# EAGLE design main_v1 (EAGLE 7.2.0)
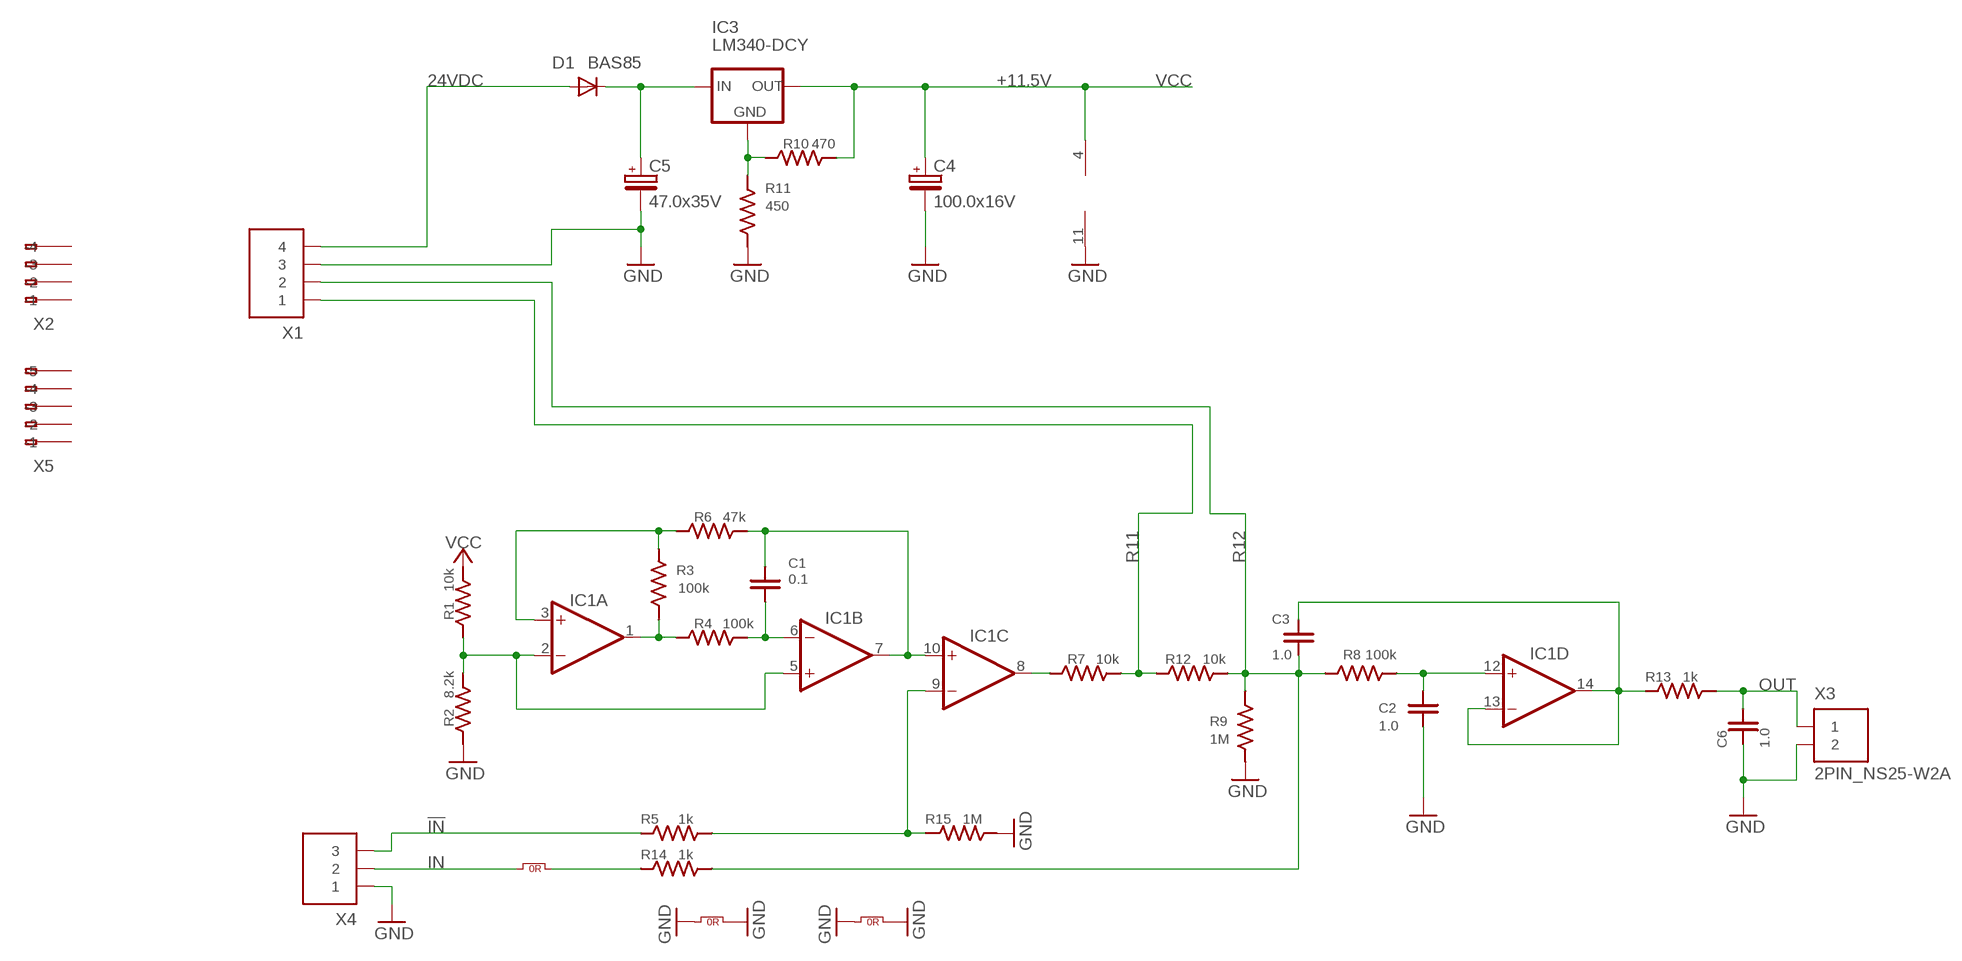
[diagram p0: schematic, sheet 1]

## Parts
C1  0.1  C/0805  [C0805]
C2  1.0  C/0805  [C0805]
C3  1.0  C/0805  [C0805]
C4  100.0x16V  CPOL-EUSANYO_SMD_C6  [SANYO-OSCON_SMD_C6]
C5  47.0x35V  CPOL-EUSANYO_SMD_C6  [SANYO-OSCON_SMD_C6]
C6  1.0  C/0805  [C0805]
D1  BAS85  DIODE-MINIMELF  [MINIMELF]
IC1  LM2902D  [SO14]
IC3  LM340-DCY  LM340MP-5V-DCY  [SOT223]
J1  0R  JUMPER  [R0805]
J2  0R  JUMPER  [R0805]
J3  0R  JUMPER  [R0805]
R1  10k  R/0805  [R0805]
R2  8.2k  R/0805  [R0805]
R3  100k  R/0805  [R0805]
R4  100k  R/0805  [R0805]
R5  1k  R/0805  [R0805]
R6  47k  R/0805  [R0805]
R7  10k  R/0805  [R0805]
R8  100k  R/0805  [R0805]
R9  1M  R/0805  [R0805]
R10  470  R/0805  [R0805]
R11  450  R/0805  [R0805]
R12  10k  R/0805  [R0805]
R13  1k  R/0805  [R0805]
R14  1k  R/0805  [R0805]
R15  1M  R/0805  [R0805]
X1  4PIN_NS25-W4A  [7395-04]
X2  233-104  [233-104]
X3  2PIN_NS25-W2A  [7395-02]
X4  3PIN_NS25-W3A  [7395-03]
X5  233-105  [233-105]

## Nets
24VDC [power]: D1.A X1.4
!IN!: R5.1 X4.3
GND: C2.1 C4.- C5.- C6.1 IC1.11(P:V-) J2.1 J2.2 J3.1 J3.2 R2.1 R9.1 R11.1 R15.1 X1.3 X3.2 X4.1
IN: J1.1 X4.2
N$1: IC1.2(A:-IN) IC1.5(B:+IN) R1.1 R2.2
N$2: IC1.3(A:+IN) R3.1 R6.1
N$3: IC1.8(C:OUT) R7.1
N$4: C1.1 IC1.6(B:-IN) R4.2
N$5: IC1.1(A:OUT) R3.2 R4.1
N$6: J1.2 R14.1
N$7: C1.2 IC1.7(B:OUT) IC1.10(C:+IN) R6.2
N$8: IC1.9(C:-IN) R5.2 R15.2
N$9: C2.2 IC1.12(D:+IN) R8.2
N$10: C3.2 IC1.13(D:-IN) IC1.14(D:OUT) R13.1
N$11: IC3.2(GND) IC3.4(GND) R10.1 R11.2
N$13 [power]: C5.+ D1.C IC3.1(IN)
OUT: C6.2 R13.2 X3.1
R11: R7.2 R12.1 X1.1
R12: C3.1 R8.1 R9.2 R12.2 R14.2 X1.2
VCC [power]: C4.+ IC1.4(P:V+) IC3.3(OUT) R1.2 R10.2
Unconnected: X2.A1(-1) X2.A2(-2) X2.A3(-3) X2.A4(-4) X2.B1(B-1) X2.B2(B-2) X2.B3(B-3) X2.B4(B-4) X5.A1(-1) X5.A2(-2) X5.A3(-3) X5.A4(-4) X5.A5(-5) X5.B1(B-1) X5.B2(B-2) X5.B3(B-3) X5.B4(B-4) X5.B5(B-5)

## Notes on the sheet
- +11.5V

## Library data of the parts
C1-C3 C6 = descreet:C
C4 C5 = rcl:CPOL-EU: POLARIZED CAPACITOR, European symbol
D1 = diode:DIODE-: DIODE
IC1 = linear:LM2902: COMPARATOR
IC3 = touch:LM340*
J1-J3 = smd-special:JUMPER
R1-R15 = descreet:R
X1 = connectors:4PIN_
X2 = con-wago:233-104: WAGO Cage Clamp
X3 = connectors:2PIN_
X4 = connectors:3PIN_
X5 = con-wago:233-105: WAGO Cage Clamp

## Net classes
0 default: clearance 0.205 mm
1 power: clearance 0.3 mm

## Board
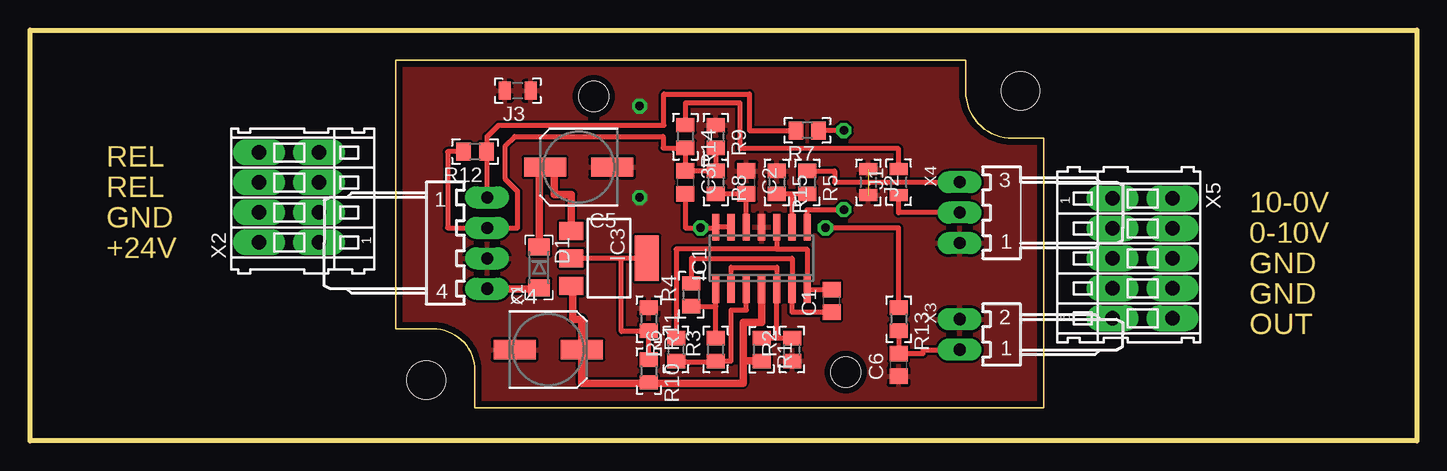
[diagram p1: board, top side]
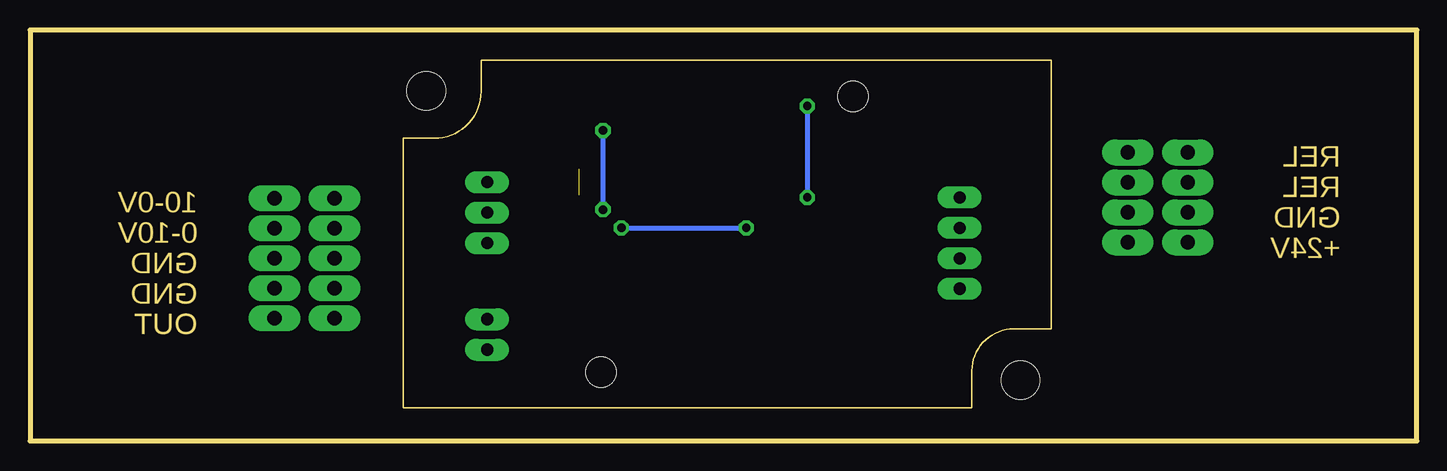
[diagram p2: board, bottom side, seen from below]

Size 115.57 x 34.29 mm. Coordinates in mm from the lower left corner, seen from the top.
Outline: 0,34.29 115.57,34.29 115.57,0 0,0 0,34.29
Copper layers (1*16): Top 0.035mm / dielectric 1.5mm / Bottom 0.035mm
Design rules "default *": minimum track width 10mil, minimum drill 24mil, track to track 8mil, track to pad 8mil, pad to pad 8mil, via to via 8mil, smd to smd 8mil, copper to edge 20mil, drill to drill 8mil, minimum pad ring 10mil, minimum via ring 8mil, stop-mask expansion 4mil, vias tented up to drill 0mil, thermal gap 10mil
Holes 3.2 mm at 33.02,5.08 82.55,29.21

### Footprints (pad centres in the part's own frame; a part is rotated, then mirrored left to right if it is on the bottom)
C0805 = smd 1.3 x 1.5: 1 -0.95,0; 2 0.95,0
SANYO-OSCON_SMD_C6 = smd 3.5 x 1.6: + 2.8,0; - -2.8,0
MINIMELF = smd 1.4 x 1.8: A 1.7,0; C -1.7,0
SO14 = smd 0.6 x 2.2: 1 -3.81,-2.6; 2 -2.54,-2.6; 3 -1.27,-2.6; 4 0,-2.6; 5 1.27,-2.6; 6 2.54,-2.6; 7 3.81,-2.6; 8 3.81,2.6; 9 2.54,2.6; 10 1.27,2.6; 11 0,2.6; 12 -1.27,2.6; 13 -2.54,2.6; 14 -3.81,2.6
SOT223 = smd 1.5 x 2: 1 -2.3,-3.15; 2 0,-3.15; 3 2.3,-3.15 | smd 3.8 x 2: 4 0,3.15
R0805 = smd 1 x 1.5: 1 -1.077,0; 2 1.077,0
R0805' = smd 1.2 x 1.5: 1 -0.95,0; 2 0.95,0
1551H = hole 2.5: 16.5,-3; 37.5,-26
7395-04 = drill 1.016 long: 1 -3.81,0; 2 -1.27,0; 3 1.27,0; 4 3.81,0
233-104 = drill 1.2 long: A1 -3.75,2.5; A2 -1.25,2.5; A3 1.25,2.5; A4 3.75,2.5; B1 -3.75,-2.5; B2 -1.25,-2.5; B3 1.25,-2.5; B4 3.75,-2.5
7395-02 = drill 1.016 long: 1 -1.27,0; 2 1.27,0
7395-03 = drill 1.016 long: 1 -2.54,0; 2 0,0; 3 2.54,0
233-105 = drill 1.2 long: A1 -5,2.5; A2 -2.5,2.5; A3 0,2.5; A4 2.5,2.5; A5 5,2.5; B1 -5,-2.5; B2 -2.5,-2.5; B3 0,-2.5; B4 2.5,-2.5; B5 5,-2.5

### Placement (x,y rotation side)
C1  66.8,11.68 90 top
C2  59.69,21.59 270 top
C3  54.61,21.59 270 top
C4  43.18,7.62 0 top
C5  45.72,22.86 180 top
C6  72.39,6.35 90 top
D1  42.42,14.48 270 top
IC1  60.96,15.24 0 top
IC3  48.26,15.24 270 top
J1  72.39,21.59 90 top
J2  69.85,21.59 270 top
J3  40.64,29.21 180 top
R1  10k  [R0805']  60.96,7.62 270 top
R2  8.2k  [R0805']  63.5,7.62 90 top
R3  100k  [R0805']  57.15,7.62 90 top
R4  100k  [R0805']  55.12,12.19 90 top
R5  1k  [R0805']  64.77,21.59 270 top
R6  47k  [R0805']  53.85,7.62 90 top
R7  10k  [R0805']  64.77,25.91 180 top
R8  100k  [R0805']  57.15,21.59 270 top
R9  1M  [R0805']  57.15,25.4 270 top
R10  470  [R0805']  51.56,5.84 270 top
R11  450  [R0805']  51.56,10.16 270 top
R12  10k  [R0805']  37.08,24.13 180 top
R13  1k  [R0805']  72.39,10.16 270 top
R14  1k  [R0805']  54.61,25.4 270 top
R15  1M  [R0805']  62.23,21.59 270 top
U$1  [1551H]  30.48,31.75 0 top
X1  38.1,16.51 270 top
X2  21.59,20.32 90 top
X3  77.47,8.89 90 top
X4  77.47,19.05 90 top
X5  92.71,15.24 270 top

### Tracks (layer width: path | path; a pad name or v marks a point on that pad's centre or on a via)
24VDC
  Top 0.406: 42.42,12.7 D1.A
  Top 0.61: X1.4 42.42,12.7
!IN!
  Top 0.406: X4.3 67.06,21.59 67.06,22.54 R5.1
GND  (via drill 0.7)  (1 unrouted)
  Bottom 0.406: v50.8,27.94 v50.8,20.32
  pour Top: 30.48,31.75 84.33,31.75 84.33,2.79 30.48,2.79
IN
  Top 0.406: X4.2 72.39,19.05 J1.1
N$1
  Top 0.406: R2.2 62.23,8.57 | IC1.2 58.42,14.48 62.23,14.48 IC1.5 62.23,8.57 | 62.23,8.57 R1.1
N$2
  Top 0.406: IC1.3 59.69,10.92 58.42,10.92 58.42,6.67 R3.1 57.15,6.6 54.61,6.6 R6.1
N$3  (via drill 0.7)
  Top 0.406: IC1.8 64.77,19.3 v67.82,19.3 | v67.82,25.91 R7.1
  Bottom 0.406: v67.82,19.3 v67.82,25.91
N$4
  Top 0.406: C1.1 63.5,10.73 IC1.6 63.5,15.24 55.12,15.24 R4.2
N$5
  Top 0.406: R3.2 57.15,11.24 | 57.15,11.24 IC1.1 | R4.1 57.15,11.24
N$6
  Top 0.406: J1.2 72.39,24.38 59.18,24.38 59.18,28.19 54.61,28.19 R14.1
N$7
  Top 0.406: IC1.10 62.23,16 | 62.23,16 64.77,16 IC1.7 C1.2 | 62.23,16 53.85,16 R6.2
N$8
  Top 0.406: R15.2 63.5,20.64 | 63.5,20.64 R5.2 | IC1.9 63.5,20.64
N$9
  Top 0.406: IC1.12 C2.2 R8.2
N$10  (via drill 0.7)
  Top 0.406: IC1.13 IC1.14 57.15,17.78 v55.88,17.78 54.61,17.78 C3.2 | R13.1 72.39,17.78 v66.29,17.78
  Bottom 0.406: v66.29,17.78 v55.88,17.78
N$11
  Top 0.406: IC3.4 49.28,15.24 | 49.28,15.24 IC3.2 | R10.1 R11.2 51.56,9.14 49.28,9.14 49.28,15.24
N$13
  Top 0.406: C5.+ 43.18,22.86 | 45.11,17.53 IC3.1
  Top 0.61: D1.C 42.42,22.36 C5.+ 43.69,22.86 43.69,20.57 45.11,20.57 IC3.1
OUT
  Top 0.406: R13.2 C6.2 74.42,7.3 74.42,7.62 X3.1
R11
  Top 0.406: X1.1 38.1,24.13 | 38.1,24.13 38.1,25.4 39.05,26.35 52.83,26.35 52.83,28.96 59.94,28.96 59.94,25.91 R7.2 | R12.1 38.1,24.13
R12
  Top 0.406: R9.2 R8.1 C3.1 R14.2 52.77,24.45 52.77,25.4 40.39,25.4 39.62,24.64 39.62,21.84 40.64,20.83 40.64,17.78 X1.2 34.8,17.78 34.8,24.13 R12.2
VCC
  Top 0.406: IC3.3 45.21,12.94
  Top 0.61: IC1.4 60.96,9.91 59.44,9.91 59.44,6.67 | 59.44,6.67 59.44,4.83 51.56,4.83 | R1.2 59.44,6.67 | 51.56,4.83 45.98,4.83 C4.+ 45.98,10.16 45.21,10.16 45.21,12.94 | R10.2 51.56,4.83

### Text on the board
Dimension: REL | REL | 10-0V | GND | 0-10V | +24V | GND | GND | OUT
